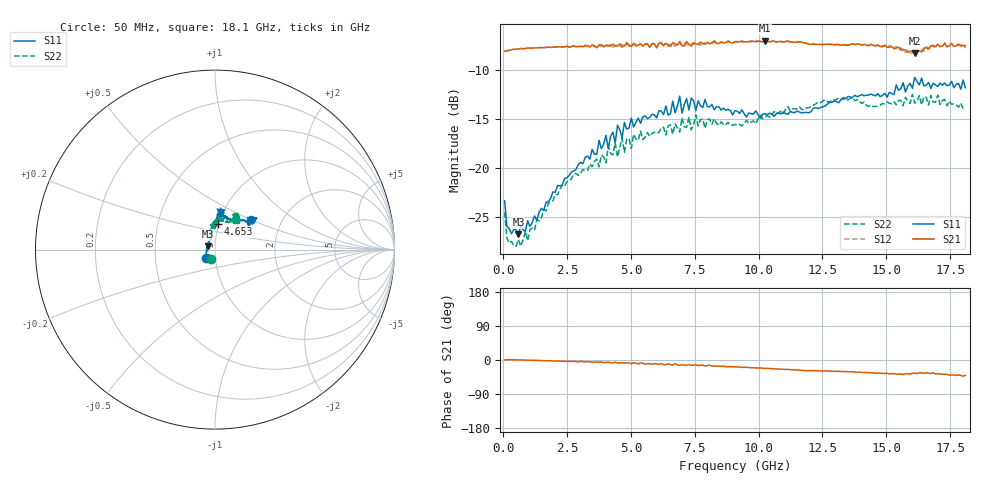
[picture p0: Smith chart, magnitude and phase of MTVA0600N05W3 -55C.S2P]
! Network Analyzer HP8720D.06.14 Serial No. US36140669
!  8 Jul 2005  13:20:24
! Frequency  S11  S21  S12  S22
# HZ  S  DB R 50
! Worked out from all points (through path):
!   201 points, 50 MHz to 18.1 GHz, reference 50 ohm
!   highest |S21| = -6.96 dB at 10.25 GHz (marker M1); lowest = -8.3 dB at 16.11 GHz (marker M2)
!   group delay of S21, straight-line fit = 6.81 ps
!   lowest |S11| = -26.8 dB at 591.5 MHz (marker M3), VSWR 1.10, Z = 46 + j1.78 ohm
!   |S11| at or under -10 dB: start of sweep to end of sweep
!   |S22| runs from -28.0 to -12.5 dB; largest |S21 - S12| = 0.023
!   S11 on the Smith chart (normalised r, x): 50 MHz: 0.90, -0.08; 4.653 GHz: 0.99, +0.29; 18.1 GHz: 1.39, +0.50
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5e7  -23.39 -136.9  -8.05 0.3  -8.07 0.3  -24.57 -113.1
2.305e8  -26.22 -177.5  -7.95 1.1  -7.95 0.9  -27.71 -177.9
5.915e8  -26.81 155.0  -7.79 0.3  -7.81 0.3  -27.36 157.1
3.1185e9  -19.57 97.9  -7.57 -4.2  -7.59 -4.6  -20.19 105.4
4.021e9  -16.66 91.6  -7.40 -6.7  -7.51 -5.7  -19.50 98.0
4.382e9  -17.44 88.2  -7.50 -5.9  -7.44 -7.7  -17.44 97.7
4.47225e9  -15.63 83.3  -7.49 -7.9  -7.37 -6.4  -18.88 101.0
4.65275e9  -16.92 83.4  -7.60 -6.7  -7.34 -8.0  -16.93 99.8
4.743e9  -15.34 86.1  -7.50 -8.3  -7.48 -7.1  -18.41 95.9
5.104e9  -15.82 88.1  -7.23 -7.8  -7.30 -9.2  -16.58 91.6
6.09675e9  -14.14 81.8  -7.22 -11.3  -7.16 -11.0  -16.34 88.9
6.7285e9  -14.36 86.0  -7.27 -10.2  -7.53 -11.6  -15.49 82.9
6.909e9  -12.64 82.6  -7.05 -14.1  -7.24 -12.3  -16.34 81.2
6.99925e9  -14.38 82.6  -7.40 -11.9  -7.49 -14.2  -14.88 82.3
7.36025e9  -12.85 76.2  -7.51 -14.4  -7.24 -13.0  -16.09 86.0
7.54075e9  -14.12 77.4  -7.29 -12.4  -7.11 -15.2  -14.57 84.6
9.075e9  -14.13 76.9  -7.06 -18.0  -7.03 -18.1  -15.54 71.6
1.024825e10  -14.43 69.1  -6.96 -22.4  -7.04 -22.1  -14.80 57.4
1.21435e10  -13.90 53.9  -7.30 -28.0  -7.25 -28.2  -13.58 59.6
1.512175e10  -12.25 35.4  -7.63 -36.7  -7.42 -36.3  -13.38 57.3
1.61145e10  -10.71 37.0  -8.26 -35.1  -7.91 -35.1  -13.37 58.4
1.81e10  -11.78 40.3  -7.48 -40.8  -7.73 -41.6  -13.91 55.3
